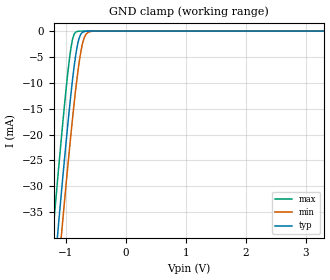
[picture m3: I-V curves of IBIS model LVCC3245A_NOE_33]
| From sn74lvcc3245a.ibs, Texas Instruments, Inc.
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[Model]   LVCC3245A_NOE_33
Model_type  Input
Vinl=0.8
Vinh=2.0
| variable   typ   min   max
C_comp   3.20pF   2.53pF   4.16pF
[Temperature Range]   40   100   -40
| Ambient temperature   25   85   -40
[Voltage range]   3.3   3   3.6
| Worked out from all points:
|   GND clamp passes 1 mA (typ) near -0.77 V on its own axis
[GND Clamp]
| LVCC3245A_NOE_33
|   Voltage   I(typ)   I(min)   I(max)
-5.5V     -655.9mA   -662.9mA   -647.3mA
-1.225V   -50.98mA   -59.27mA   -40.34mA
-1.145V   -40.42mA   -48.72mA   -29.76mA
-1.12V    -37.16mA   -45.46mA   -26.51mA
-1.08V    -32.02mA   -40.29mA   -21.41mA
-1.06V    -29.48mA   -37.73mA   -18.91mA
-965mV    -17.86mA   -25.9mA    -7.899mA
-885mV    -9.107mA   -16.56mA   -1.488mA
-780mV    -1.473mA   -6.233mA   -17.17uA
-715mV    -205.6uA   -2.13mA    -809.4nA
-640mV    -15.54uA   -338.4uA   -23.72nA
3.3V      6.304pA    9.26pA     5.93pA
